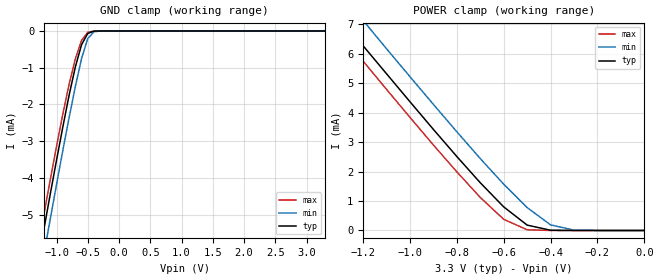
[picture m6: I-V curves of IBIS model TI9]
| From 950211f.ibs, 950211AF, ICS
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|   Model TI9
[Model]   TI9
Model_type   Input
Polarity   Non-Inverting
Vinl = 800.00mV
Vinh =   2.00V
C_comp   5.50pF   5.00pF   6.00pF
[Temperature Range]   27.00   70.00   0.00
[Voltage Range]   3.30V   3.00V   3.70V
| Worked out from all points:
|   GND clamp passes 1 mA (typ) near -0.70 V on its own axis
|   POWER clamp passes 1 mA (typ) near -0.62 V on its own axis
[GND_clamp]
| voltage   I(typ)   I(min)   I(max)
-3.3V     -25.94mA   -26.62mA   -25.53mA
-1.3V     -6.33mA    -7.02mA    -5.92mA
-1.2V     -5.38mA    -6.06mA    -4.98mA
-1.1V     -4.44mA    -5.12mA    -4.05mA
-900mV    -2.62mA    -3.26mA    -2.27mA
-800mV    -1.76mA    -2.37mA    -1.46mA
-700mV    -985.4uA   -1.52mA    -763uA
-600mV    -374.8uA   -752.5uA   -256.1uA
-500mV    -64.68uA   -205.4uA   -34.13uA
-400mV    -4.39uA    -20.4uA    -1.64uA
-300mV    -161.1nA   -1.12uA    -40.9nA
3.3V      122.6pA    11.86uA    89.8pA
[POWER_clamp]
| voltage   I(typ)   I(min)   I(max)
-3.3V     26.92mA    27.75mA    26.41mA
-1.4V     8.21mA     9.06mA     7.68mA
-1.3V     7.24mA     8.09mA     6.71mA
-1.2V     6.27mA     7.13mA     5.75mA
-1.1V     5.32mA     6.17mA     4.79mA
-800mV    2.51mA     3.35mA     1.99mA
-700mV    1.62mA     2.44mA     1.12mA
-600mV    800.4uA    1.57mA     378.2uA
-500mV    182.1uA    776.2uA    24.18uA
-400mV    7.5uA      190.6uA    384.6nA
-300mV    162nA      11.86uA    5.68nA
0V        122.7pA    241.2pA    133.4pA
